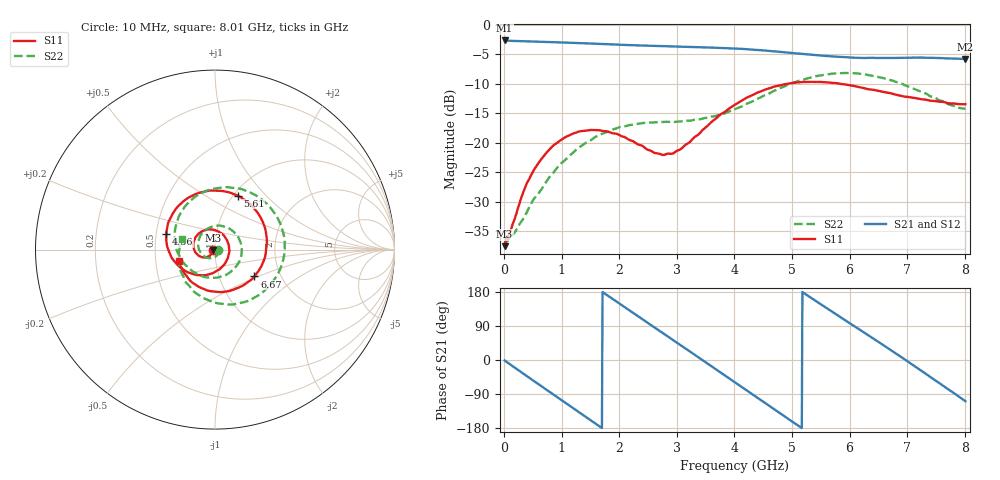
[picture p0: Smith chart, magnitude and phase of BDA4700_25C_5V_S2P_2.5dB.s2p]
!Agilent Technologies,E5071B,MY42404982,A.09.10
!Date: Mon Oct 20 13:27:09 2025
!Data & Calibration Information:
!Freq	S11:SOLT2(ON)	S21:SOLT2(ON)	S12:SOLT2(ON)	S22:SOLT2(ON)
# Hz S RI R 50
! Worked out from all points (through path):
!   801 points, 10 MHz to 8.01 GHz, reference 50 ohm
!   highest |S21| = -2.61 dB at 10 MHz (marker M1); lowest = -5.8 dB at 8.01 GHz (marker M2)
!   group delay of S21, straight-line fit = 286 ps
!   lowest |S11| = -37.6 dB at 10 MHz (marker M3), VSWR 1.03, Z = 48.7 - j0.175 ohm
!   |S11| at or under -10 dB: start of sweep to 4.905 GHz; 5.844 GHz to end of sweep
!   |S22| runs from -36.8 to -8.1 dB; largest |S21 - S12| = 0.0054
!   S11 on the Smith chart (normalised r, x): 10 MHz: 0.97, -0.00; 4.56 GHz: 0.57, +0.11; 5.61 GHz: 1.04, +0.70; 6.67 GHz: 1.47, -0.47; 8.01 GHz: 0.66, -0.09
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1e7  -0.0131 -0.0018  0.74 -0.0158  0.74 -0.0167  0.0156 -0.00158
3.3e8  -0.0238 -0.029  0.5936 -0.4229  0.5935 -0.4237  0.0169 -0.0148
7.1e8  -0.0662 -0.0433  0.178 -0.6968  0.1778 -0.6973  -0.00673 -0.0443
1.02e9  -0.1063 -0.0185  -0.2235 -0.6752  -0.224 -0.6751  -0.0549 -0.0409
1.35e9  -0.1199 0.0369  -0.5603 -0.4221  -0.5606 -0.4226  -0.0931 0.0167
1.64e9  -0.0944 0.0863  -0.688 -0.0804  -0.6881 -0.0804  -0.0745 0.0876
1.93e9  -0.042 0.112  -0.6266 0.2729  -0.6269 0.2733  -0.00207 0.1312
2.32e9  0.0341 0.0908  -0.2956 0.6033  -0.2955 0.604  0.1117 0.0921
2.68e9  0.0758 0.0283  0.1272 0.652  0.1273 0.6517  0.1483 -0.0212
3.36e9  0.0162 -0.1148  0.6421 0.0974  0.6428 0.0968  -0.00753 -0.157
3.67e9  -0.0701 -0.1429  0.5878 -0.257  0.5876 -0.2587  -0.102 -0.1341
4.01e9  -0.1795 -0.11  0.3236 -0.543  0.3239 -0.5421  -0.1817 -0.0642
4.56e9  -0.2718 0.087  -0.2726 -0.5408  -0.2726 -0.5413  -0.2165 0.138
4.96e9  -0.1896 0.2565  -0.5401 -0.2162  -0.5407 -0.218  -0.1078 0.2962
5.35e9  -0.00844 0.3291  -0.5322 0.1719  -0.5329 0.1708  0.1063 0.3437
5.61e9  0.1255 0.3009  -0.3924 0.3785  -0.3928 0.3792  0.254 0.2842
6.12e9  0.2828 0.1001  0.0417 0.5264  0.0443 0.5267  0.3889 -0.00214
6.67e9  0.2195 -0.1496  0.4531 0.2677  0.4534 0.2667  0.2108 -0.2721
6.68e9  0.2164 -0.1534  0.4573 0.2594  0.4585 0.2587  0.2056 -0.2747
7.24e9  -0.00303 -0.234  0.4672 -0.247  0.4664 -0.2477  -0.0835 -0.2574
7.63e9  -0.1369 -0.1749  0.1898 -0.4868  0.1892 -0.4879  -0.1967 -0.1093
8.01e9  -0.2029 -0.0634  -0.1655 -0.4883  -0.1648 -0.4889  -0.1852 0.0587
